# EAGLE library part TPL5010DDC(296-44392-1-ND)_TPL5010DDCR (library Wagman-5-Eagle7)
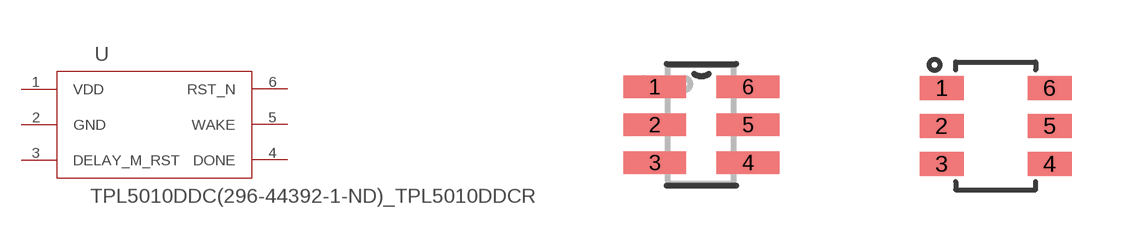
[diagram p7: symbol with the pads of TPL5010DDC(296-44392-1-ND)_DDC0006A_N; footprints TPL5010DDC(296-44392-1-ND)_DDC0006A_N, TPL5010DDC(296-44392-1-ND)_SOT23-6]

Designator prefix U

## TPL5010DDC(296-44392-1-ND)_TPL5010DDCR (COMPTYPE: IC; MANUFACTURER: Texas Instruments; MOUNTTYPE: SMT; PACKAGEREFERENCE: DDC0006A; PARTNUMBER: TPL5010DDC; PIN_COUNT: 6; REFDES: RefDes; ROHS: Y; TYPE: TYPE; VALUE: Value)  [TPL5010DDC(296-44392-1-ND)_DDC0006A_N]
1  VDD  pwr
2  GND  pwr
3  DELAY_M_RST  in
4  DONE  in
5  WAKE  out
6  RST_N  out

## TPL5010DDC(296-44392-1-ND)_TPL5010DDCRDDC0006A_L (COMPTYPE: IC; MANUFACTURER: Texas Instruments; MOUNTTYPE: SMT; PACKAGEREFERENCE: DDC0006A; PARTNUMBER: TPL5010DDC; PIN_COUNT: 6; REFDES: RefDes; ROHS: Y; TYPE: TYPE; VALUE: Value)  [TPL5010DDC(296-44392-1-ND)_SOT23-6]
Pads as for TPL5010DDC(296-44392-1-ND)_DDC0006A_N

## TPL5010DDC(296-44392-1-ND)_TPL5010DDCRDDC0006A_M (COMPTYPE: IC; MANUFACTURER: Texas Instruments; MOUNTTYPE: SMT; PACKAGEREFERENCE: DDC0006A; PARTNUMBER: TPL5010DDC; PIN_COUNT: 6; REFDES: RefDes; ROHS: Y; TYPE: TYPE; VALUE: Value)  [TPL5010DDC(296-44392-1-ND)_DDC0006A_M]
Pads as for TPL5010DDC(296-44392-1-ND)_DDC0006A_N

## Footprint TPL5010DDC(296-44392-1-ND)_DDC0006A_N (pad centres in mm)
smd 1.575 x 0.559: 1 -1.168,0.95; 2 -1.168,0; 3 -1.168,-0.95; 4 1.168,-0.95; 5 1.168,0; 6 1.168,0.95

## Footprint TPL5010DDC(296-44392-1-ND)_SOT23-6 (pad centres in mm)
smd 1.1 x 0.6: 1 -1.35,0.95; 2 -1.35,0; 3 -1.35,-0.95; 4 1.35,-0.95; 5 1.35,0; 6 1.35,0.95

## Footprint TPL5010DDC(296-44392-1-ND)_DDC0006A_M (pad centres in mm)
smd 1.88 x 0.61: 1 -1.118,0.95; 2 -1.118,0; 3 -1.118,-0.95; 4 1.118,-0.95; 5 1.118,0; 6 1.118,0.95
